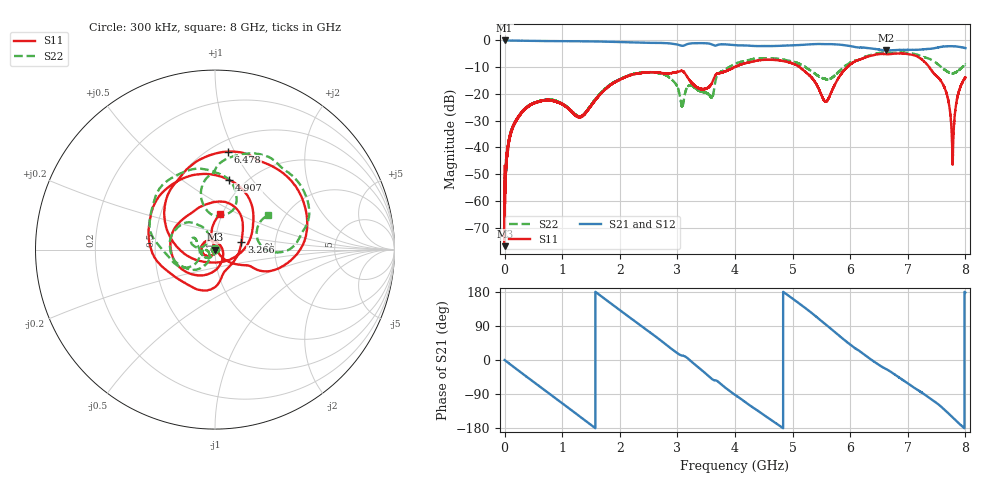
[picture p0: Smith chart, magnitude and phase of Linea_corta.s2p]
#  HZ  S  DB  R  50.00
! Rohde & Schwarz ZVA/B
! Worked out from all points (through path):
!   30000 points, 300 kHz to 8 GHz, reference 50 ohm
!   highest |S21| = 0.01 dB at 566.7 kHz (marker M1); lowest = -3.7 dB at 6.63 GHz (marker M2)
!   group delay of S21, straight-line fit = 310 ps
!   lowest |S11| = -76.9 dB at 1.1 MHz (marker M3), VSWR 1.00, Z = 50 - j0.00249 ohm
!   |S11| at or under -10 dB: start of sweep to 3.99 GHz; 5.124 GHz to 5.946 GHz (822.2 MHz wide, 14.9 % of centre); 7.374 GHz to end of sweep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
!   |S22| runs from -70.8 to -4.5 dB; largest |S21 - S12| = 0.0031
!   S11 on the Smith chart (normalised r, x): 300 kHz: 1.00, +0.01; 3.266 GHz: 1.34, +0.12; 4.907 GHz: 0.84, +0.78; 6.478 GHz: 0.60, +0.95; 8 GHz: 0.97, +0.41
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300000  -46.98 111.6  0.00 -0.1  -0.00 -0.1  -52.19 83.9
566665.6  -57.12 109.6  0.01 -0.1  0.00 -0.1  -59.39 165.1
1099997  -76.90 -170.0  0.00 -0.1  -0.00 -0.1  -67.18 -178.0
1.205662e8  -33.78 -101.2  -0.05 -14.1  -0.05 -14.1  -33.32 -99.7
3.888317e8  -24.93 -140.4  -0.13 -44.8  -0.13 -44.8  -24.89 -127.2
8.512298e8  -22.64 155.2  -0.24 -97.3  -0.24 -97.3  -22.34 -168.0
1.333628e9  -28.27 20.9  -0.30 -152.2  -0.31 -152.2  -28.44 -149.4
2.085625e9  -13.81 -143.1  -0.65 122.0  -0.65 122.0  -13.72 -153.4
2.666956e9  -12.04 143.3  -0.91 56.8  -0.92 56.8  -12.19 152.8
3.080554e9  -11.37 75.3  -1.99 11.8  -1.99 11.8  -24.84 138.7
3.266153e9  -16.24 17.0  -1.04 -7.2  -1.04 -7.1  -17.13 151.8
3.588552e9  -16.33 -75.0  -1.38 -48.7  -1.39 -48.7  -21.26 -179.0
4.000283e9  -9.90 -165.5  -1.76 -92.0  -1.77 -92.0  -8.70 165.9
4.90668e9  -8.02 78.9  -1.89 172.3  -1.89 172.3  -7.42 87.6
5.333611e9  -13.94 15.4  -1.40 123.8  -1.40 123.8  -11.56 64.8
5.582677e9  -22.82 -95.3  -1.37 92.8  -1.38 92.8  -14.44 83.7
6.47814e9  -5.18 82.3  -3.32 -10.7  -3.32 -10.8  -4.76 68.1
6.629606e9  -5.12 65.5  -3.74 -24.4  -3.74 -24.5  -4.51 55.3
6.666939e9  -5.14 62.5  -3.69 -27.6  -3.69 -27.6  -4.57 52.8
7.553335e9  -14.47 -27.5  -2.49 -119.9  -2.49 -120.0  -9.43 -2.7
7.776534e9  -45.89 8.6  -2.15 -151.1  -2.15 -151.1  -12.24 15.1
8e9  -13.80 81.8  -2.85 178.1  -2.85 178.1  -8.98 32.5
